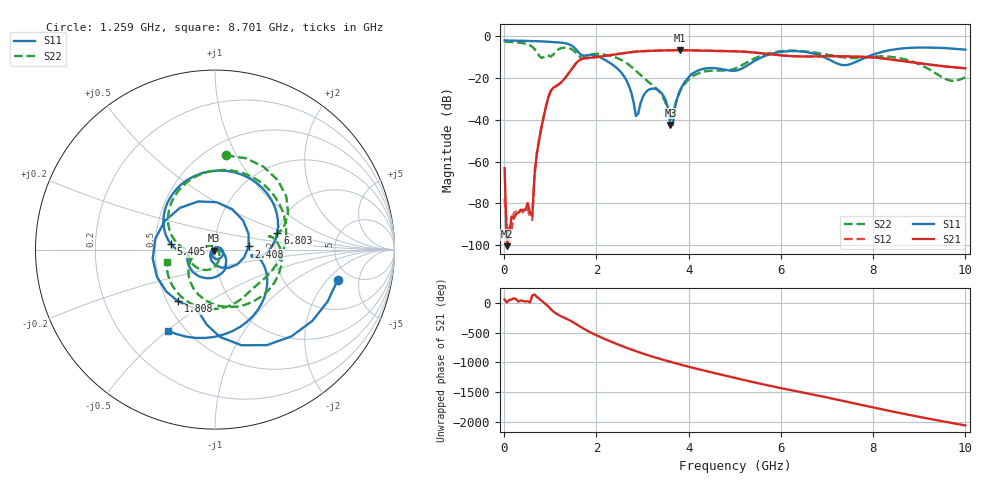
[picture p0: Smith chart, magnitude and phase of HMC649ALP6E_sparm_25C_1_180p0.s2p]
!Analog Devices Inc..
!GaAs MMIC 6-BIT DIGITAL PHASE SHIFTER, 3 - 6 GHz
!Filename: HMC649ALP6E_sparm_25C_1_180p0.s2p
!  :25C = 25degC
!  :_1_ = Sn1
!  :_180p0  = 180.0 state
!Device type:
!2 Port Calibration to sma connectors
!Phase Shifter:  0.000
!	Vss= -5V, Vdd= +5V , control Voltage = 0/ +5V
!Freq	S11	S11	S21	S21	S12	S12	S22	S22
! GHz	Mag dB	Degrees	Mag dB	Degrees	Mag dB	Degrees	Mag dB	Degrees
# GHZ S DB R 50.0
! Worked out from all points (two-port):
!   201 points, 10 MHz to 10 GHz, reference 50 ohm
!   highest |S21| = -6.61 dB at 3.806 GHz (marker M1); lowest = -100.6 dB at 59.95 MHz (marker M2)
!   |S21| within 3 dB of the highest: 2.111 GHz to 6.427 GHz (4.317 GHz wide, 101 % of centre); 6.717 GHz to 7.511 GHz (794.2 MHz wide, 11.2 % of centre)
!   lowest |S11| = -42.5 dB at 3.606 GHz (marker M3), VSWR 1.02, Z = 49.6 - j0.64 ohm
!   |S11| at or under -10 dB: 2.073 GHz to 5.586 GHz (3.513 GHz wide, 91.7 % of centre); 6.935 GHz to 7.851 GHz (916.1 MHz wide, 12.4 % of centre)
!   |S22| runs from -40.2 to -2.6 dB; largest |S21 - S12| = 0.00099
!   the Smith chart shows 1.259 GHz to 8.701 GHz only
!   S11 on the Smith chart (normalised r, x): 1.259 GHz: 3.93, -2.63; 1.808 GHz: 0.57, -0.37; 2.408 GHz: 1.46, +0.05; 5.405 GHz: 0.60, +0.04; 6.803 GHz: 2.00, +0.43; 8.701 GHz: 0.40, -0.50
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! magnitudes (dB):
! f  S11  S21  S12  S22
! 10 MHz  -1.9  -63.2  -77.9  -2.6
! 59.95 MHz  -2.0  -100.6  -91.0  -2.6
! 609.4 MHz  -2.2  -86.1  -88.1  -5.0
! 709.3 MHz  -2.3  -56.2  -56.1  -7.5
! 909.1 MHz  -2.5  -33.4  -33.4  -9.1
! 1.259 GHz  -3.0  -21.5  -21.5  -5.5
! 1.708 GHz  -9.2  -10.7  -10.7  -10.2
! 1.808 GHz  -9.0  -10.4  -10.3  -9.2
! 2.408 GHz  -14.5  -8.6  -8.6  -10.0
! 2.707 GHz  -23.8  -7.7  -7.6  -13.7
! 2.857 GHz  -38.2  -7.3  -7.3  -16.5
! 3.357 GHz  -26.0  -6.8  -6.8  -26.3
! 3.606 GHz  -42.5  -6.6  -6.6  -40.2
! 3.806 GHz  -26.3  -6.6  -6.6  -26.6
! 4.256 GHz  -15.9  -6.8  -6.8  -17.4
! 5.005 GHz  -16.5  -7.2  -7.1  -15.4
! 5.405 GHz  -12.1  -7.7  -7.7  -10.8
! 6.703 GHz  -8.2  -9.6  -9.6  -7.6
! 6.803 GHz  -8.9  -9.6  -9.6  -8.0
! 8.352 GHz  -6.7  -11.0  -10.9  -9.7
! 8.701 GHz  -5.6  -12.0  -12.0  -11.1
! 10 GHz  -6.3  -15.3  -15.3  -19.6
